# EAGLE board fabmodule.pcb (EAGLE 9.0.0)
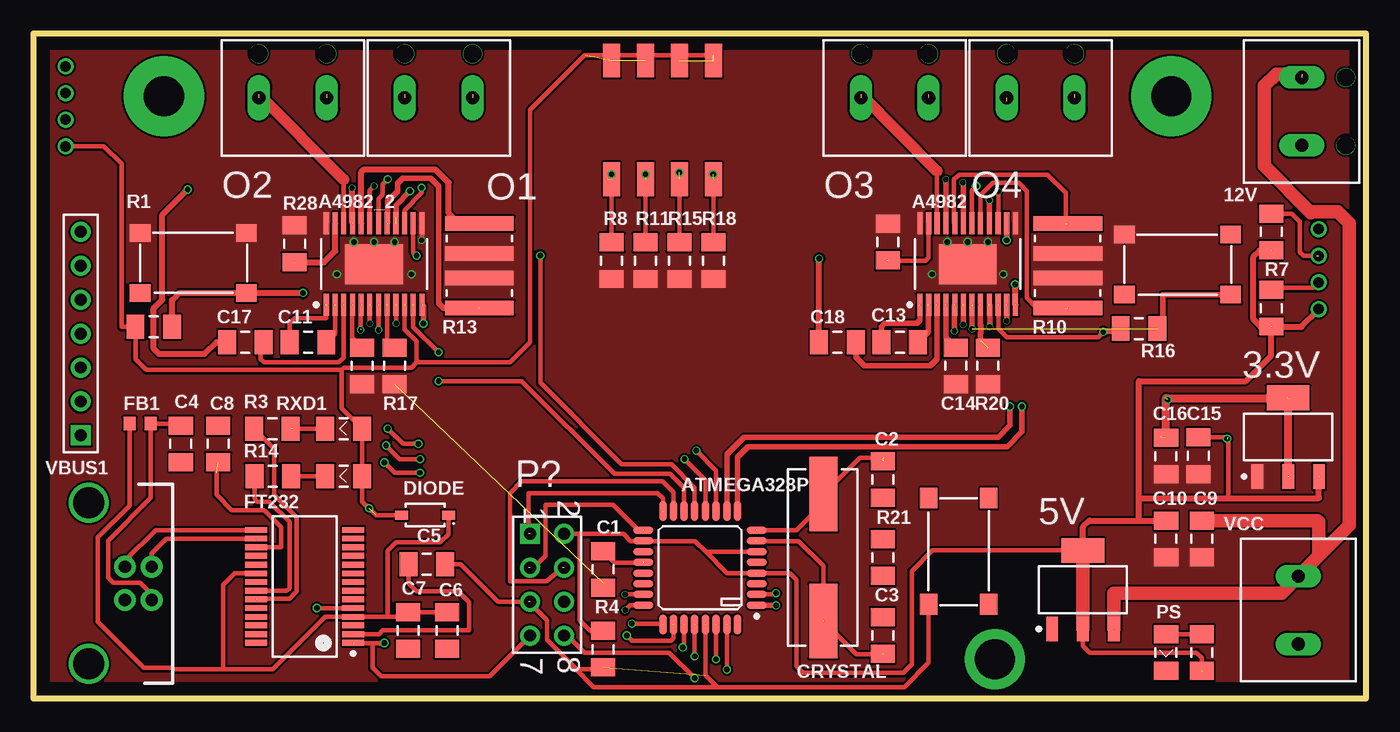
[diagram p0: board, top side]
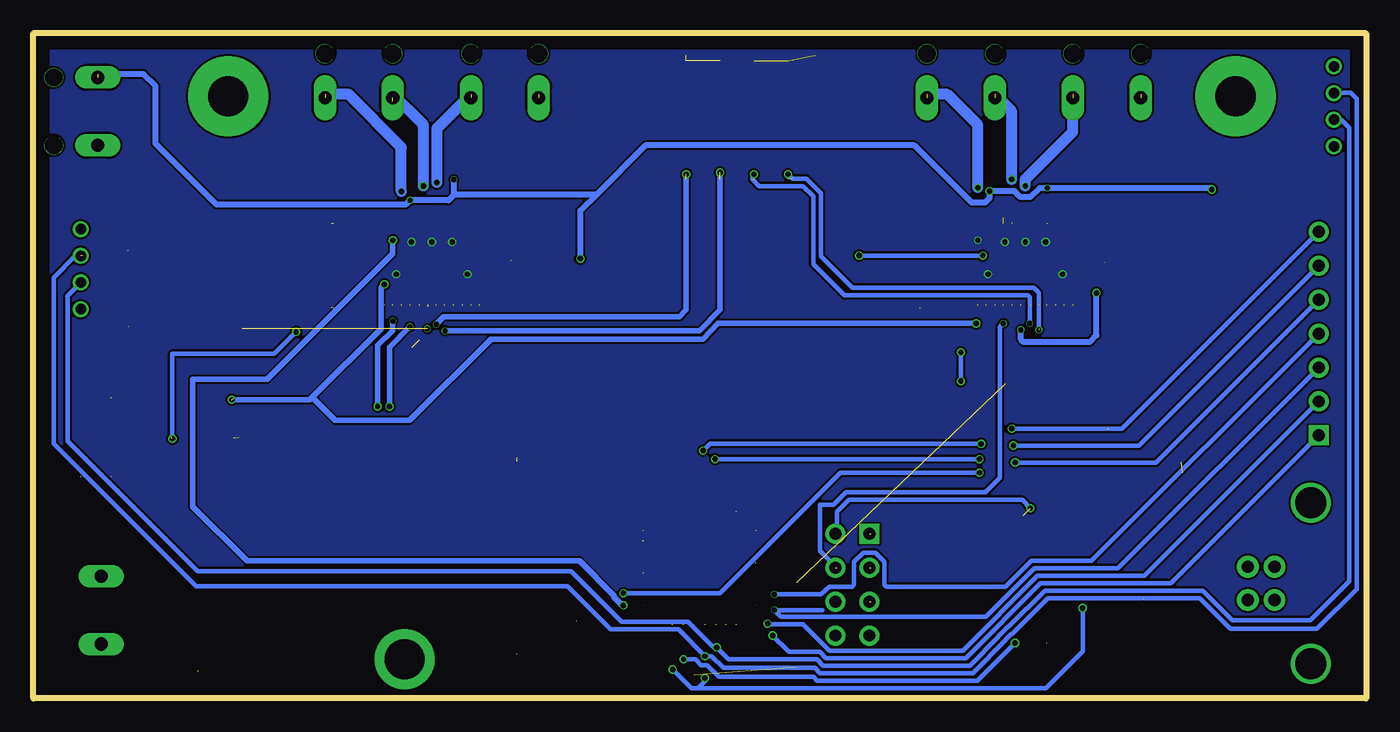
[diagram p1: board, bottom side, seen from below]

Size 99.82 x 49.78 mm. Coordinates in mm from the lower left corner, seen from the top.
Outline: 0,0 99.82,0 99.82,49.78 0,49.78 0,0
Copper layers (1*16): Top 0.035mm / dielectric 1.5mm / Bottom 0.035mm
Design rules "FabModule": minimum track width 6mil, minimum drill 0.35mm, track to track 6mil, track to pad 6mil, pad to pad 6mil, via to via 6mil, smd to smd 6mil, copper to edge 40mil, drill to drill 6mil, minimum pad ring 0mil, minimum via ring 0mil, stop-mask expansion 4mil, vias tented up to drill 0mil, thermal gap 10mil

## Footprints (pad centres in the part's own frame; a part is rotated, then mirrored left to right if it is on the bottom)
SOT223_1PRIMARY = smd 1.854 x 0.889: 1 -2.946,2.311; 2 -2.946,0; 4 -2.946,-2.311 | smd 1.854 x 3.2: 3 2.946,0
2PIN_1PRIMARY = drill 0.991 pad 1.702 long: 1 0,0; 2 5.08,0 | drill 1.346 pad 1.397: 3 5.08,-3.302; 4 0,-3.302
TSSOP-24_1PRIMARY = smd 1.651 x 0.381: 1 -3.048,3.581; 2 -3.048,2.921; 3 -3.048,2.286; 4 -3.048,1.626; 5 -3.048,0.965; 6 -3.048,0.33; 7 -3.048,-0.33; 8 -3.048,-0.965; 9 -3.048,-1.626; 10 -3.048,-2.286; 11 -3.048,-2.921; 12 -3.048,-3.581; 13 3.048,-3.581; 14 3.048,-2.921; 15 3.048,-2.286; 16 3.048,-1.626; 17 3.048,-0.965; 18 3.048,-0.33; 19 3.048,0.33; 20 3.048,0.965; 21 3.048,1.626; 22 3.048,2.286; 23 3.048,2.921; 24 3.048,3.581 | smd 2.997 x 4.318: 25 0,0
TSSOP-24_2PRIMARY = smd 1.651 x 0.381: 1 -3.048,3.581; 2 -3.048,2.921; 3 -3.048,2.286; 4 -3.048,1.626; 5 -3.048,0.965; 6 -3.048,0.33; 7 -3.048,-0.33; 8 -3.048,-0.965; 9 -3.048,-1.626; 10 -3.048,-2.286; 11 -3.048,-2.921; 12 -3.048,-3.581; 13 3.048,-3.581; 14 3.048,-2.921; 15 3.048,-2.286; 16 3.048,-1.626; 17 3.048,-0.965; 18 3.048,-0.33; 19 3.048,0.33; 20 3.048,0.965; 21 3.048,1.626; 22 3.048,2.286; 23 3.048,2.921; 24 3.048,3.581 | smd 2.997 x 4.318: 25 0,0
TQFP-32_1PRIMARY = smd 1.499 x 0.559: 1 -4.242,2.794; 2 -4.242,2.007; 3 -4.242,1.194; 4 -4.242,0.406; 5 -4.242,-0.406; 6 -4.242,-1.194; 7 -4.242,-2.007; 8 -4.242,-2.794; 17 4.242,-2.794; 18 4.242,-2.007; 19 4.242,-1.194; 20 4.242,-0.406; 21 4.242,0.406; 22 4.242,1.194; 23 4.242,2.007; 24 4.242,2.794 | smd 0.559 x 1.499: 9 -2.794,-4.242; 10 -2.007,-4.242; 11 -1.194,-4.242; 12 -0.406,-4.242; 13 0.406,-4.242; 14 1.194,-4.242; 15 2.007,-4.242; 16 2.794,-4.242; 25 2.794,4.242; 26 2.007,4.242; 27 1.194,4.242; 28 0.406,4.242; 29 -0.406,4.242; 30 -1.194,4.242; 31 -2.007,4.242; 32 -2.794,4.242
CAPC1206_1PRIMARY = smd 1.346 x 1.803: 1 -1.372,0; 2 1.372,0
HC49/US_1PRIMARY = smd 5.588 x 2.108: 1 -4.75,0; 2 4.75,0
HDR1X7_1PRIMARY = drill 0.889 pad 1.499 square: 1 0,0 | drill 0.889 pad 1.499: 2 2.54,0; 3 5.08,0; 4 7.62,0; 5 10.16,0; 6 12.7,0; 7 15.24,0
SOD-123_1PRIMARY = smd 0.965 x 0.66: 1 -1.753,0; 2 1.753,0
IND0603_1PRIMARY = smd 0.914 x 0.991: 1 -0.787,0; 2 0.787,0
TSSOP-28_1PRIMARY = smd 1.651 x 0.432: 1 -3.632,4.216; 2 -3.632,3.581; 3 -3.632,2.921; 4 -3.632,2.286; 5 -3.632,1.626; 6 -3.632,0.965; 7 -3.632,0.33; 8 -3.632,-0.33; 9 -3.632,-0.965; 10 -3.632,-1.626; 11 -3.632,-2.286; 12 -3.632,-2.921; 13 -3.632,-3.581; 14 -3.632,-4.216; 15 3.632,-4.216; 16 3.632,-3.581; 17 3.632,-2.921; 18 3.632,-2.286; 19 3.632,-1.626; 20 3.632,-0.965; 21 3.632,-0.33; 22 3.632,0.33; 23 3.632,0.965; 24 3.632,1.626; 25 3.632,2.286; 26 3.632,2.921; 27 3.632,3.581; 28 3.632,4.216
GROVE90_1PRIMARY = drill 0.787 pad 1.194: 1 -2.997,0; 2 -0.991,0; 3 0.991,0; 4 2.997,0
DIPSWITCH-04-SMD_1PRIMARY = smd 1.27 x 2.54: 1 -3.81,4.445; 2 -1.27,4.445; 3 1.27,4.445; 4 3.81,4.445; 5 3.81,-4.445; 6 1.27,-4.445; 7 -1.27,-4.445; 8 -3.81,-4.445
HDR2X4_1PRIMARY = drill 0.889 pad 1.499 square: 1 0,0 | drill 0.889 pad 1.499: 2 0,2.54; 3 2.54,0; 4 2.54,2.54; 5 5.08,0; 6 5.08,2.54; 7 7.62,0; 8 7.62,2.54
LED1206_1PRIMARY = smd 1.346 x 1.803: 1 -1.372,0; 2 1.372,0
BUTTON_1PRIMARY = smd 1.549 x 1.295: 1 0,0; 2 7.95,0; 3 0,-4.496; 4 7.95,-4.496
RESC1206_1PRIMARY = smd 1.346 x 1.803: 1 -1.372,0; 2 1.372,0
RESC1020_1PRIMARY = smd 1.092 x 5.156: 1 -1.118,0; 2 1.118,0
USB_B_1PRIMARY = drill 0.914 pad 1.626: 1 -1.245,0; 2 -1.245,2.007; 3 1.245,0; 6 1.245,2.007 | drill 2.311 pad 2.997: 4 -6.02,-2.718; 5 6.02,-2.718
2PIN_2PRIMARY = drill 0.991 pad 1.702 long: 1 0,0; 2 5.08,0

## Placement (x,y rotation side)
3.3V  VREG  [SOT223_1PRIMARY]  93.98,19.56 90 top
5V  VREG  [SOT223_1PRIMARY]  78.61,8.13 90 top
12V  [2PIN_1PRIMARY]  95,41.4 90 top
A4982  A4982  [TSSOP-24_1PRIMARY]  69.98,32.51 90 top
A4982_2  A4982  [TSSOP-24_2PRIMARY]  25.53,32.51 90 top
ATMEGA328P  ATmega328P-AU  [TQFP-32_1PRIMARY]  49.94,9.78 180 top
C1  100nf  [CAPC1206_1PRIMARY]  42.67,9.65 90 top
C2  22pf  [CAPC1206_1PRIMARY]  63.63,16.38 90 top
C3  22pf  [CAPC1206_1PRIMARY]  63.63,4.7 270 top
C4  10nF  [CAPC1206_1PRIMARY]  11.05,19.05 90 top
C5  100nF  [CAPC1206_1PRIMARY]  29.46,10.03 180 top
C6  100nf  [CAPC1206_1PRIMARY]  30.99,5.08 90 top
C7  4.7uF  [CAPC1206_1PRIMARY]  28.07,5.08 90 top
C8  100nf  [CAPC1206_1PRIMARY]  13.84,19.05 270 top
C9  10uf  [CAPC1206_1PRIMARY]  87.5,11.94 90 top
C10  0.1uf  [CAPC1206_1PRIMARY]  84.84,11.94 90 top
C11  0.1uf  [CAPC1206_1PRIMARY]  20.57,26.67 180 top
C12  0.22uf  [CAPC1206_1PRIMARY]  24.64,24.89 90 top
C13  0.1uf  [CAPC1206_1PRIMARY]  64.9,26.67 180 top
C14  0.22uf  [CAPC1206_1PRIMARY]  69.09,24.89 90 top
C15  10uf  [CAPC1206_1PRIMARY]  87.25,18.16 90 top
C16  0.1uf  [CAPC1206_1PRIMARY]  84.84,18.14 90 top
C17  0.1uf  [CAPC1206_1PRIMARY]  15.88,26.67 180 top
C18  0.1uf  [CAPC1206_1PRIMARY]  60.22,26.67 180 top
CRYSTAL  16Mhz  [HC49/US_1PRIMARY]  59.18,10.54 270 top
D/A  Header_7  [HDR1X7_1PRIMARY]  3.56,19.68 90 top
DIODE  SS1P3L  [SOD-123_1PRIMARY]  29.34,13.72 180 top
FB1  FerriteBead  [IND0603_1PRIMARY]  8,20.57 180 top
FT232  FT232RL-Reel  [TSSOP-28_1PRIMARY]  20.32,8.38 180 top
I2C  [GROVE90_1PRIMARY]  96.27,32.13 90 top
I2C_  [GROVE90_1PRIMARY]  2.41,44.32 90 top
MS  [DIPSWITCH-04-SMD_1PRIMARY]  47.12,43.31 180 top
O1  [2PIN_1PRIMARY]  32.89,44.96 180 top
O2  [2PIN_1PRIMARY]  21.97,44.96 180 top
O3  [2PIN_1PRIMARY]  67.06,44.96 180 top
O4  [2PIN_1PRIMARY]  77.98,44.96 180 top
P?  Header_4X2  [HDR2X4_1PRIMARY]  37.21,12.32 270 top
PS  [LED1206_1PRIMARY]  84.84,3.43 270 top
R1  [BUTTON_1PRIMARY]  8,34.85 0 top
R2  [BUTTON_1PRIMARY]  81.71,34.72 0 top
R3  270  [RESC1206_1PRIMARY]  17.91,20.19 180 top
R4  1k  [RESC1206_1PRIMARY]  42.67,3.68 270 top
R5  330  [RESC1206_1PRIMARY]  87.5,3.43 270 top
R6  4.7K  [RESC1206_1PRIMARY]  92.71,29.21 90 top
R7  4.7K  [RESC1206_1PRIMARY]  92.71,34.92 90 top
R8  20k  [RESC1206_1PRIMARY]  43.31,32.77 90 top
R9  .2  [RESC1020_1PRIMARY]  77.47,34.42 90 top
R10  .2  [RESC1020_1PRIMARY]  77.47,30.35 270 top
R11  20k  [RESC1206_1PRIMARY]  45.85,32.77 90 top
R12  .2  [RESC1020_1PRIMARY]  33.4,34.42 90 top
R13  .2  [RESC1020_1PRIMARY]  33.4,30.35 270 top
R14  270  [RESC1206_1PRIMARY]  17.93,16.64 180 top
R15  20k  [RESC1206_1PRIMARY]  48.39,32.77 90 top
R16  20k  [RESC1206_1PRIMARY]  82.8,27.69 180 top
R17  20k  [RESC1206_1PRIMARY]  27.05,24.89 270 top
R18  20k  [RESC1206_1PRIMARY]  50.93,32.77 90 top
R19  20k  [RESC1206_1PRIMARY]  9.02,27.81 0 top
R20  20k  [RESC1206_1PRIMARY]  71.5,24.89 270 top
R21  1M  [RESC1206_1PRIMARY]  63.63,10.54 90 top
R28  20k  [RESC1206_1PRIMARY]  19.56,34.04 90 top
R29  20k  [RESC1206_1PRIMARY]  64.01,34.16 90 top
RESET  [BUTTON_1PRIMARY]  71.55,14.99 270 top
RXD1  [LED1206_1PRIMARY]  23.24,20.19 180 top
TXD1  [LED1206_1PRIMARY]  23.24,16.64 180 top
VBUS1  USB-B  [USB_B_1PRIMARY]  6.86,8.61 270 top
VCC  Header_2  [2PIN_2PRIMARY]  94.74,4.06 90 top

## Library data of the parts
3.3V 5V 12V A4982 A4982_2 ATMEGA328P C1-C18 CRYSTAL D/A DIODE FB1 FT232 I2C I2C_ MS O1-O4 P? PS R1-R21 R28 R29 RESET RXD1 TXD1 VBUS1 VCC = FabModule

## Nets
1: ATMEGA328P.26 D/A.1
2: ATMEGA328P.25 D/A.2
3: ATMEGA328P.24 D/A.3
3.3V: 3.3V.2 3.3V.3 A4982.12 A4982_2.12 C16.2
3V3: C8.2 FT232.17
4: ATMEGA328P.23 D/A.4
5: ATMEGA328P.2 D/A.5
5V: 3.3V.4 A4982.10 A4982_2.10 C10.2 C15.2 DIODE.2 MS.5 MS.6 MS.7 MS.8 R5.2 R6.1 R7.1 R16.2 R19.1
6: ATMEGA328P.12 D/A.6
7: ATMEGA328P.11 D/A.7
12V: 5V.4 12V.2 A4982.16 A4982.21 A4982_2.16 A4982_2.21 C9.2 C17.2 C18.2 VCC.2
D1: A4982_2.14 ATMEGA328P.13
D2: A4982.14 ATMEGA328P.1
ENA: A4982_2.23 R28.1
ENA2: A4982.23 R29.1
GND: 3.3V.1 A4982.13 A4982.24 A4982.25 A4982_2.13 A4982_2.24 A4982_2.25 C9.1 C10.1 C12.1 C14.1 C15.1 C16.1 R1.1 R1.2 R2.1 R8.1 R9.1 R10.1 R11.1 R12.1 R13.1 R15.1 R17.2 R18.1 R20.2 R28.2 R29.2
MISO: ATMEGA328P.16 P?.1
MOSI: A4982_2.9 ATMEGA328P.15 P?.4
MS1: A4982_2.5 MS.4 R8.2
MS2: A4982_2.6 MS.3 R11.2
MS3: A4982.5 MS.2 R15.2
MS4: A4982.6 MS.1 R18.2
NETA4982_1: A4982.1 C13.2
NETA4982_2: A4982.2 C13.1
NETA4982_2_1: A4982_2.1 C11.2
NETA4982_2_2: A4982_2.2 C11.1
NETA4982_2_3: A4982_2.3 C17.1
NETA4982_2_4: A4982_2.4 C12.2
NETA4982_2_8: A4982_2.8 R17.1
NETA4982_2_15: A4982_2.15 O1.1
NETA4982_2_17: A4982_2.17 R13.2
NETA4982_2_18: A4982_2.18 O1.2
NETA4982_2_19: A4982_2.19 O2.1
NETA4982_2_20: A4982_2.20 R12.2
NETA4982_2_22: A4982_2.22 O2.2
NETA4982_3: A4982.3 C18.1
NETA4982_4: A4982.4 C14.2
NETA4982_8: A4982.8 R20.1
NETA4982_15: A4982.15 O4.1
NETA4982_17: A4982.17 R10.2
NETA4982_18: A4982.18 O4.2
NETA4982_19: A4982.19 O3.1
NETA4982_20: A4982.20 R9.2
NETA4982_22: A4982.22 O3.2
NETATMEGA328P_7: ATMEGA328P.7 C3.2 CRYSTAL.2
NETATMEGA328P_8: ATMEGA328P.8 C2.2 CRYSTAL.1
NETATMEGA328P_20: ATMEGA328P.20 C1.2
NETC4_2: C4.2 FB1.1 VBUS1.6
NETC5_2: C5.2 FT232.2
NETFT232_15: FT232.15 VBUS1.1
NETFT232_16: FT232.16 VBUS1.2
NETFT232_22: FT232.22 R14.2
NETFT232_23: FT232.23 R3.2
NETPS_1: R5.1
NETR2_1: R3.1
R1: A4982_2.7 R1.4 R19.2
R2: A4982.7 R2.4 R16.1
RESET: ATMEGA328P.29 C5.1 P?.5 R4.2 RESET.4
RXD: ATMEGA328P.30 FT232.1 P?.7
SCK: ATMEGA328P.17 P?.3
SCL: ATMEGA328P.28 R7.2
SDA: ATMEGA328P.27 R6.2
SL2: A4982.9 ATMEGA328P.10
ST1: A4982_2.11 ATMEGA328P.14
ST2: A4982.11 ATMEGA328P.9
TXD: ATMEGA328P.31 FT232.5 P?.8
VUSB: C6.2 C7.2 DIODE.1 FB1.2 FT232.4 FT232.20

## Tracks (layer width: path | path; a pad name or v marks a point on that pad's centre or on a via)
1  (via drill 0.4 pad 0.61)  (1 unrouted)
  Top 0.356: 47.93,5.51 47.93,4.5 47.75,4.32 44.83,4.32 v44.45,4.7
  Bottom 0.356: v44.45,4.7 43.23,3.48 40.92,3.48 40.46,3 29.97,3 24.38,8.61 14.63,8.61 D/A.1
2  (via drill 0.4 pad 0.61)  (1 unrouted)
  Top 0.356: 47.14,5.51 47.07,5.59 v44.83,5.59
  Bottom 0.356: v44.83,5.59 44.78,5.54 42.19,5.54 40.21,3.56 30.2,3.56 24.61,9.17 16.61,9.17 D/A.2
3  (via drill 0.4 pad 0.51)  (1 unrouted)
  Top 0.356: v44.32,6.6 44.7,6.96 45.69,6.96
  Bottom 0.356: 40.72,6.6 v44.32,6.6 43.81,6.1 28.47,6.1 24.84,9.73 18.59,9.73 D/A.3
3.3V  (via drill 0.4 pad 0.61)  (6 unrouted)
  Top 0.406: v29.21,28.07 29.21,29.34 29.11,29.44
  Top 0.457: 73.56,29.44 73.56,30.96
  Top 0.61: 84.45,19.53 84.84,19.91 84.84,22.48 93.95,22.48 93.98,22.43 93.98,16.59 | v73.53,30.99 73.56,30.96
  Bottom 0.406: v29.21,28.07 48.54,28.07 49.68,26.9 65.53,26.9 71.63,20.83 77.22,20.83 78.94,22.53 | 78.94,22.53 73.79,27.69 73.79,30.73 v73.53,30.99 | 78.94,22.53 79.12,22.35 v84.96,22.35
3V3  (1 unrouted)
  Top 0.356: 13.72,16.89 13.72,15.24 14.86,14.1 17.27,14.1 18.54,12.8 18.54,11.3 FT232.17
4  (via drill 0.4 pad 0.51)
  Top 0.356: v44.32,7.77 ATMEGA328P.23
  Bottom 0.356: v44.32,7.77 40.82,7.77 40.21,8.36 38.48,8.36 38.35,8.48 38.35,10.24 37.67,10.9 36.75,10.9 36.07,10.24 36.07,8.48 35.94,8.36 27,8.36 25.07,10.29 20.57,10.29 D/A.4
5  (via drill 0.4 pad 0.61)
  Top 0.356: v55.63,7.87 55.52,7.77 ATMEGA328P.2 | v26.29,17.65 27.05,16.89 v28.96,16.89
  Bottom 0.356: v55.63,7.87 48.39,7.87 39.37,16.89 v28.96,16.89 | D/A.5 15.75,17.65 v26.29,17.65
5V  (via drill 0.4 pad 0.61)  (14 unrouted)
  Top 0.356: C15.2 89.51,19.53 89.51,14.99 | 50.93,48.13 41.28,48.13 37.21,44.07 37.21,26.67 35.69,25.15 28.7,25.15 | 54.18,9.37 56.67,9.37 57.15,8.89 57.15,2.41 57.66,1.91 65.15,1.91 65.79,2.54 65.79,9.52 67.33,11.07 78.61,11.07 | 40.89,12.32 40.89,5.84 41.68,5.05 42.67,5.05 | 2.41,41.33 5.26,41.33 6.6,40 6.6,27.81 R19.1 7.64,25.38 8.43,24.59 23.09,24.59 | 27.81,29.44 27.81,27.61 28.7,26.72 28.7,25.15 | 72.26,29.44 72.26,27.69 72.9,27.05 79.76,27.05 v80.14,27.43 81.18,27.43 R16.2 | 23.09,24.59 23.09,21.72 24.61,20.19 24.61,14.73 25.65,13.72 DIODE.2 | 96.27,14.99 96.29,14.99 | 23.09,24.59 23.27,24.76 28.32,24.76 28.7,25.15 | 87.5,2.03 87.5,3.05 87.12,3.43 79.12,3.43 78.61,3.94 78.61,5.16 | 40.89,12.32 44.2,12.32 44.73,11.76 49.55,11.76 50.37,10.97 | 39.62,12.32 40.89,12.32 | 50.37,10.97 51.97,9.37 54.13,9.37 | 50.37,10.97 54.13,10.97
  Top 0.457: 96.29,14.99 96.29,16.59 | 92.71,33.53 91.85,33.53 91.39,33.07 91.39,28.37 91.92,27.81 92.71,27.81 | 96.27,29.11 94.97,27.81 92.71,27.81 | 92.71,27.81 92.71,25.65 90.8,23.75 82.8,23.75 82.8,14.99 | 82.8,14.99 89.51,14.99 96.27,14.99 | 82.8,13.31 82.8,14.99 | 82.8,13.31 C10.2 | 82.8,13.31 79.1,13.31 78.61,12.83 78.61,11.07
  Top 1: 78.61,5.16 78.61,11.07
  Bottom 0.356: 39.62,12.32 39.62,13.97 38.73,14.86 25.76,14.86 v25.15,14.22 | v80.14,27.43 81.79,25.78 89.41,25.78 v89.41,19.43
6  (via drill 0.4 pad 0.61)
  Top 0.356: v26.42,18.92 27.43,17.91 v28.96,17.91 | v48.77,17.91 50.34,16.33 ATMEGA328P.12
  Bottom 0.356: D/A.6 17.02,18.92 v26.42,18.92 | v28.96,17.91 v48.77,17.91
7  (via drill 0.4 pad 0.61)
  Top 0.356: v26.54,20.19 27.69,19.05 v28.83,19.05 | v49.66,18.54 51.13,17.04 ATMEGA328P.11
  Bottom 0.356: D/A.7 18.29,20.19 v26.54,20.19 | v28.83,19.05 49.15,19.05 v49.66,18.54
12V  (via drill 0.4 pad 0.51, 0.4 pad 0.61)  (5 unrouted)
  Top 0.406: v28.19,37.97 28.19,37.95 27.15,36.91 27.15,35.97 | v68.33,38.84 68.35,38.81 A4982.21 | A4982.16 v71.6,37.29
  Top 0.457: C18.2 v58.85,32.92 | v11.56,38.1 9.65,36.19 9.65,29.85 9.02,29.21 9.02,26.16 9.4,25.78 12.83,25.78 13.72,26.67 C17.2 | 23.88,35.58 v23.88,38.2
  Top 1: 96.29,10.67 98.55,12.95 98.55,35.56 97.69,36.42 95.73,36.42 95.68,36.37 92.2,39.88 92.2,45.85 93.09,46.74 95,46.74 | 96.29,10.67 VCC.2 93.5,7.87 80.92,7.87 80.92,5.16 | 96.29,10.67 96.29,13.21 96.16,13.31 C9.2
  Bottom 0.457: 57.66,37.69 58.85,36.53 v58.85,32.92 | 57.66,37.69 53.97,41.4 33.83,41.4 29.54,37.11 28.55,37.11 28.19,37.47 v28.19,37.97 26.34,37.97 25.88,37.52 25.17,37.52 24.46,38.2 v23.88,38.2 11.68,38.2 v11.56,38.1 | 57.66,37.69 68.33,37.69 | 95,46.74 91.57,46.74 90.68,45.85 90.68,41.53 86.11,36.96 71.96,36.96 v71.6,37.29 68.73,37.29 68.33,37.69 | 68.33,37.69 v68.33,38.84
D1  (via drill 0.4 pad 0.61)
  Top 0.356: ATMEGA328P.13 49.53,15.75 47.78,17.53 44.07,17.53 37.97,23.62 v37.97,33.15 | v28.7,33.15 28.45,33.38 A4982_2.14
  Bottom 0.356: v28.7,33.15 v37.97,33.15
D2  (via drill 0.4 pad 0.61)  (1 unrouted)
  Top 0.406: 54.18,6.96 v55.63,6.96 | v72.9,34.29 A4982.14
  Bottom 0.406: v55.63,6.96 55.73,6.96 56.34,7.57 56.34,7.67 58.93,10.29 83.82,10.29 87.88,14.35 87.88,23.88 82.3,23.88 72.9,33.27 v72.9,34.29
ENA  (1 unrouted)
  Top 0.457: 19.56,32.64 21.74,32.64 22.61,33.5 A4982_2.23
ENA2  (1 unrouted)
  Top 0.356: A4982.23 67.06,33 66.83,32.77 64.01,32.77
GND  (via drill 0.4 pad 0.51, 0.4 pad 0.61)  (1 unrouted)
  Top 0.356: v29.08,34.29 29.11,34.29 A4982_2.13 | 42.67,8.25 42.67,8.64
  other vias: 71.5,34.16 69.98,34.16 68.45,34.16 67.31,31.75 72.64,31.75 24,34.16 25.53,34.16 27.05,34.16 28.32,31.75 22.73,31.75
  pour Bottom (no thermals): 0,-0.01 0,49.77 99.82,49.77 99.82,-0.01
  pour Top (no thermals): 0.25,0.51 0.25,49.63 99.67,49.63 99.67,0.1 0.25,0.1
MISO  (2 unrouted)
  Top 0.356: 47.14,13.97 47.14,14.96 46.74,15.37 37.08,15.37 37.08,12.32
MOSI  (via drill 0.4 pad 0.51)  (3 unrouted)
  Top 0.356: 47.93,13.97 ATMEGA328P.15 47.93,15.42 47.12,16.26 36.58,16.26 35.69,15.37 35.69,8.76 38.43,8.76 39.62,9.78 | v27.18,28.07 27.15,28.09 27.15,29.44
  Bottom 0.356: v27.18,28.07 27.43,27.81 27.43,16.51 28.52,15.42 38.96,15.42 39.9,14.48 40.89,14.48 40.89,11.05 39.62,9.78
MS1  (via drill 0.4 pad 0.51, 0.4 pad 0.61)  (3 unrouted)
  Top 0.356: R8.2 v43.31,39.24 | 24.51,27.69 24.51,29.41 24.56,29.44
  Bottom 0.356: v24.51,27.58 24.51,30.35 24.89,30.73 38.48,30.73 40.84,33.1 40.84,37.82 41.94,38.91 42.98,38.91 v43.31,39.24 43.43,39.24
MS2  (via drill 0.4 pad 0.51, 0.4 pad 0.61)  (2 unrouted)
  Top 0.356: R11.2 v45.85,39.24 | v25.2,28.07 25.2,29.44
  Bottom 0.356: v25.2,28.07 25.2,30.02 25.35,30.18 39.06,30.18 41.4,32.51 41.4,37.59 42.16,38.35 45.47,38.35 45.97,38.86 45.97,39.12 v45.85,39.24
MS3  (via drill 0.4 pad 0.51, 0.4 pad 0.61)  (3 unrouted)
  Top 0.356: R15.2 48.39,39.24
  Top 0.406: v68.99,27.51 68.99,29.44 69.01,29.44
  Bottom 0.406: v68.99,27.51 49.94,27.51 48.39,29.08 v48.39,39.37
MS4  (via drill 0.4 pad 0.51, 0.4 pad 0.61)  (2 unrouted)
  Top 0.356: R18.2 v50.93,39.24
  Top 0.406: v69.65,27.99 69.65,29.44
  Bottom 0.406: v69.65,27.99 69.09,28.57 51.44,28.57 50.93,29.08 v50.93,39.24
NETA4982_1  (1 unrouted)
  Top 0.406: 66.4,29.44 66.4,28.3 66.17,28.07 63.75,28.07 63.52,27.81 C13.2
NETA4982_2  (1 unrouted)
  Top 0.406: 67.06,29.44 67.06,27.43 C13.1
NETA4982_2_1  (1 unrouted)
  Top 0.356: 21.95,29.44 21.95,28.45 19.56,28.45 19.2,28.07 C11.2
NETA4982_2_2  (1 unrouted)
  Top 0.356: 22.61,29.44 22.61,27.31 C11.1
NETA4982_2_3  (1 unrouted)
  Top 0.356: 23.24,29.44 23.24,25.5 22.86,25.15 17.27,25.15 17.02,25.4 17.02,26.42 C17.1
NETA4982_2_4  (1 unrouted)
  Top 0.356: C12.2 23.88,27 23.88,29.44 23.9,29.44
NETA4982_2_8  (1 unrouted)
  Top 0.356: R17.1 26.49,26.8 26.49,29.44 26.54,29.41
NETA4982_2_15  (via drill 0.4 pad 0.61)  (1 unrouted)
  Top 0.356: v29.08,38.23 29.08,37.85 27.81,36.55 A4982_2.15
  Bottom 0.813: v29.08,38.23 29.08,42.93 31.37,45.21 32.89,45.21
NETA4982_2_17  (2 unrouted)
  Top 0.406: 26.52,35.56 26.52,37.21 27.28,37.95 27.28,38.56 27.66,38.94 29.74,38.94 30.35,38.35 30.35,29.59 30.71,29.21 33.4,29.21
NETA4982_2_18  (via drill 0.4 pad 0.61)  (1 unrouted)
  Top 0.356: v26.54,38.86 26.16,38.48 26.16,37.72 25.86,37.39 A4982_2.18
  Bottom 0.813: v26.54,38.86 26.54,43.94 27.81,45.21
NETA4982_2_19  (via drill 0.4 pad 0.51)  (1 unrouted)
  Top 0.356: v25.53,38.35 25.2,38.02 A4982_2.19
  Bottom 0.813: v25.53,38.35 25.53,38.86 21.97,42.42 21.97,45.21
NETA4982_2_20
  Top 0.457: A4982_2.20 24.56,39.42 24.77,39.6 30.1,39.6 31.11,38.61 31.11,36.32 31.9,35.53 R12.2
NETA4982_2_22  (1 unrouted)
  Top 0.356: A4982_2.22 23.24,38.84
  Top 0.813: 16.89,45.21 23.24,38.84
NETA4982_3  (1 unrouted)
  Top 0.406: 67.69,29.44 67.69,25.4 67.18,24.89 62.23,24.89 61.59,25.53 C18.1
NETA4982_4  (1 unrouted)
  Top 0.406: 68.35,29.44 68.35,27 C14.2
NETA4982_8  (2 unrouted)
  Top 0.406: 70.94,26.8 70.94,27.36 70.97,27.38 70.97,27.92 70.94,27.94 70.94,29.44
NETA4982_15  (via drill 0.4 pad 0.51)  (1 unrouted)
  Top 0.356: A4982.15 v72.26,37.95
  Bottom 0.813: v72.26,37.95 72.26,41.25 76.2,45.21 77.98,45.21
NETA4982_17  (1 unrouted)
  Top 0.356: A4982.17 70.94,37.67 71.86,38.58 73.81,38.58 74.42,37.97 74.42,29.97 75.16,29.21 77.34,29.21
NETA4982_18  (via drill 0.4 pad 0.61)  (2 unrouted)
  Top 0.356: v70.61,38.35 70.31,38.02 A4982.18 | 72.9,44.7 72.9,45.21
  Bottom 0.813: v70.61,38.35 70.61,42.93 72.9,45.21
NETA4982_19  (via drill 0.4 pad 0.51)  (1 unrouted)
  Top 0.406: v69.6,38.61 69.65,38.53 A4982.19
  Bottom 0.813: v69.6,38.61 69.6,42.67 67.06,45.21
NETA4982_20  (1 unrouted)
  Top 0.356: A4982.20 68.96,35.58 68.96,38.86 69.34,39.22 75.95,39.22 77.34,37.85 77.34,35.53
NETA4982_22  (1 unrouted)
  Top 0.356: A4982.22 67.69,39.47
  Top 0.813: 61.98,45.21 67.69,39.47
NETATMEGA328P_7  (3 unrouted)
  Top 0.356: 54.13,11.76 57.3,11.76 59.18,9.91 59.18,5.77 61.65,3.3 63.63,3.3
NETATMEGA328P_8  (2 unrouted)
  Top 0.356: 54.13,12.57 57.15,12.57 59.18,14.61 CRYSTAL.1 61.9,18.01 63.63,18.01
NETATMEGA328P_20  (1 unrouted)
  Top 0.356: C1.2 43.51,10.16 45.75,10.16
NETC4_2
  Top 0.356: VBUS1.6 8.87,7.77 8,8.64 5.97,8.64 5.59,9.02 5.59,11.81 8.79,15.01 FB1.1 10.9,20.57 C4.2
NETC5_2
  Top 0.356: 24,4.85 FT232.2 25.88,4.8 26.16,5.08 32.64,5.08 32.64,7.19 31.83,8 28.7,8 28.09,8.61 C5.2
NETFT232_15
  Top 0.356: FT232.15 9.17,12.6 6.86,10.29 VBUS1.1
NETFT232_16  (1 unrouted)
  Top 0.356: 16.69,11.94 9.93,11.94 8.87,10.87 VBUS1.2
NETFT232_22
  Top 0.356: R14.2 16.56,14.93 16.76,14.73 17.65,14.73 19.18,13.21 19.18,8.25 18.97,8.05 FT232.22
NETFT232_23  (1 unrouted)
  Top 0.356: R3.2 18.03,18.67 18.03,15.24 19.74,13.54 19.74,8 19.18,7.44 16.69,7.44 16.69,7.39
NETPS_1
  Top 0.356: 84.84,4.8 R5.1
NETR2_1  (1 unrouted)
  Top 0.356: 19.41,20.19 21.87,20.19
NETR3_1
  Top 0.356: 19.3,16.64 21.87,16.64
R1  (via drill 0.4 pad 0.51, 0.4 pad 0.61)  (1 unrouted)
  Top 0.356: v25.86,27.58 25.86,29.44
  Top 0.457: v20.19,30.35 R1.4 10.92,30.35 10.39,29.82 R19.2
  Bottom 0.457: v20.19,30.35 20.19,27.18 20.7,26.67 25.65,26.67 25.86,26.85 v25.86,27.58
R2  (via drill 0.4 pad 0.51)  (2 unrouted)
  Top 0.406: v70.31,27.66 70.31,29.36 | R16.1 84.58,28.07 84.58,30.23 R2.4
RESET  (4 unrouted)
  Top 0.356: 40.69,2.16 40.64,2.16 41.96,0.84 65.23,0.84 67.06,2.67 RESET.4 | 40.69,2.16 42.52,2.16 42.67,2.29 | 40.69,2.16 38.48,4.37 38.48,5.84 37.08,7.24 34.8,7.24 32,10.03 C5.1 | 51.18,0.89 50.34,1.73 50.34,5.56
RXD  (via drill 0.4 pad 0.61)  (2 unrouted)
  Top 0.356: 23.95,4.14 25.4,4.14 | 25.4,4.14 v26.29,4.14 | P?.7 34.16,1.65 26.04,1.65 25.4,2.29 25.4,4.14 | v51.13,2.92 51.13,5.51
  Bottom 0.356: v51.13,2.92 50.24,2.92 49.81,2.46 49.35,2.46 48.46,1.6 41.4,1.6 41.15,1.32 29.11,1.32 v26.29,4.14
S$1  (via drill 3 pad 4.5)
  other vias: 72.01,2.92
S$2  (via drill 3 pad 5.99)
  other vias: 85.22,45.08
S$3  (via drill 3 pad 5.99)
  other vias: 9.78,45.08
SCK  (2 unrouted)
  Top 0.356: 45.75,12.57 45.34,12.57 43.43,14.48 38.35,14.48 38.35,10.67 37.47,9.78 37.08,9.78
SCL  (via drill 0.4 pad 0.61)  (2 unrouted)
  Top 0.356: v49.53,3.15 49.53,5.51 | R7.2 94.26,36.3 94.87,35.69 94.87,33.4 95.15,33.12 96.27,33.12
  Bottom 0.356: 2.41,45.34 1.14,45.34 0.71,44.91 0.71,8.18 3.68,5.21 10.16,5.21 12.45,7.49 23.85,7.49 26.49,4.83 26.57,4.83 26.97,4.42 26.97,4.37 29.44,1.88 40.92,1.88 41.3,2.29 48.13,2.29 49.02,3.15 v49.53,3.15 51.51,5.16 56.59,5.16 59.82,8.38 87.63,8.38 98.3,19.05 98.3,31.5 96.67,33.12 96.14,33.12
SDA  (via drill 0.4 pad 0.61)  (2 unrouted)
  Top 0.356: 48.74,5.51 48.74,3.89 v48.64,3.81 48.64,3.86 | 96.27,31.11 95.86,30.73 92.86,30.73 R6.2
  Bottom 0.356: 2.41,43.33 1.85,43.33 1.27,42.72 1.27,8.76 4.19,5.84 10.01,5.84 12.22,8.05 24.08,8.05 26.75,5.39 26.8,5.39 27.53,4.65 27.53,4.6 29.69,2.44 40.69,2.44 41.15,2.92 47.75,2.92 v48.64,3.81 48.87,3.81 50.77,5.71 55.75,5.71 59.56,9.52 87.5,9.52 97.26,19.25 97.26,30.07 97.28,30.1 96.27,31.11
SL2  (via drill 0.4 pad 0.51, 0.4 pad 0.61)  (1 unrouted)
  Top 0.406: v71.63,27.81 71.63,29.41 71.6,29.44 | v73.15,21.84 73.15,20.45 72.26,19.56 53.21,19.56 51.94,18.26 ATMEGA328P.10
  Bottom 0.406: v71.63,27.81 73.15,26.29 v73.15,21.84
ST1  (via drill 0.4 pad 0.61)  (1 unrouted)
  Top 0.356: v30.35,23.75 36.58,23.75 43.51,16.82 47.7,16.82 48.74,15.77 ATMEGA328P.14 | v30.35,25.91 28.45,27.79 28.45,29.44
  Bottom 0.356: v30.35,23.75 v30.35,25.91
ST2  (via drill 0.4 pad 0.51, 0.4 pad 0.61)  (1 unrouted)
  Top 0.406: v72.9,28.25 72.9,29.44 | v74.04,21.84 74.04,19.94 72.95,18.82 53.52,18.82 52.73,18.06 ATMEGA328P.9
  Bottom 0.406: v72.9,28.25 72.9,27.53 74.04,26.42 v74.04,21.84
TXD  (via drill 0.4 pad 0.61)  (1 unrouted)
  Top 0.356: v49.53,1.52 47.62,3.43 41.28,3.43 40,4.7 P?.8 | v51.94,2.16 51.94,5.51 | v21.23,6.76 FT232.5
  Bottom 0.356: v51.94,2.16 50.55,0.76 50.04,0.76 | 50.04,0.76 24,0.76 21.23,3.5 v21.23,6.76 | 50.04,0.76 49.53,1.27 v49.53,1.52
VUSB
  Top 0.356: 14.22,2.16 10.54,2.16 10.41,2.29 8.26,2.29 4.83,5.71 4.83,12.07 7.21,14.43 FB1.2 | 14.22,2.16 17.91,2.16 21.84,6.1 FT232.4 26.54,6.1 | 14.22,2.16 14.22,8.51 15.06,9.35 FT232.20 | DIODE.1 31.09,12.27 30.48,11.68 27.18,11.68 26.54,11.05 26.54,6.1 | 26.54,6.1 27.71,6.1 C7.2 C6.2 31.39,6.45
